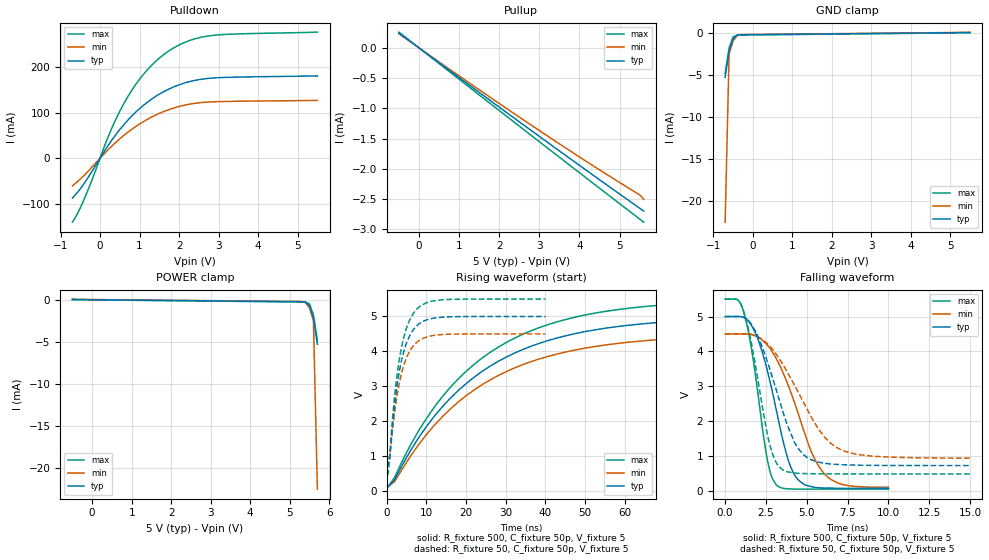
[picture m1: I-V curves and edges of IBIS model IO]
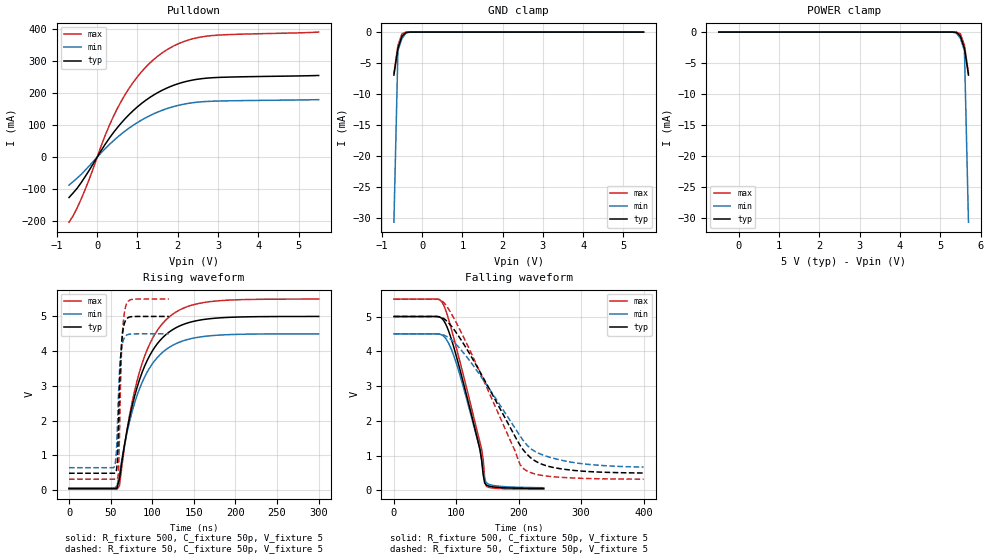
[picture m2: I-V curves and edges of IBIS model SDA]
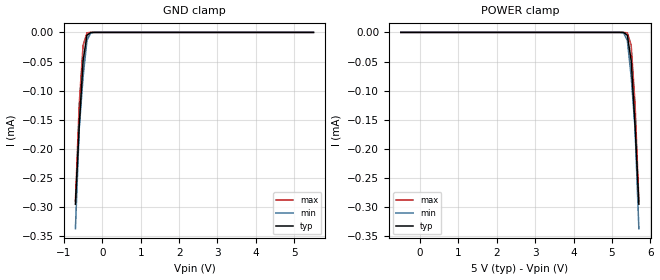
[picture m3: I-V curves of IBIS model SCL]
[IBIS Ver]   3.2
[Comment Char]   |_char
| VDD Nom: 5v, Min: 4.5v, Max: 5.5v
[File name]   pca9673_5v.ibs
[File Rev]   1
[Date]   08-25-2008
[Source]
[Notes]
[Disclaimer]
(C) Copyright 2007 NXP Semiconductors
All rights reserved
NXP Semiconductors (NXP) does not warrant that this model and any other
accompanying information (Model) accurately or fully represents the
operating characteristics and specifications of the semiconductor
products to which the Model relates.  Moreover, the Model is furnished
on an "as is" and with "all faults" basis, and without support or
warranty of any kind.  NXP disclaims all warranties, whether expressed
or implied or statutory, including without limitation all implied
warranties of non-infringement, merchantability and fitness for any
purpose, and those arising from a course of dealing or usage of trade.
NXP does not convey any license under its or any third party's patents,
copyrights or other intellectual property or proprietary rights.
You and your company assume any and all risks and liability arising out
of the application or use of the Model.
In no event shall NXP be liable for any direct, indirect, special,
consequential or incidental damages, however caused, whether in
warranty, contract or tort (including negligence), strict liability or
other legal theory, including, without limitation, for lost profits,
business interruption, or corruption or loss of data or information,
arising out of or in connection with the use of or the inability to use
the Model, even if NXP has been advised of the possibility of such
damages.
NXP provides the Model as a courtesy to our customers. You and your
company shall not distribute, convey, sell, or give the Model to anyone
else without receiving prior written permission from NXP.
NXP reserves the right to make changes without notice to the Model to
improve reliability, function, or design.
Please be aware that your receipt and subsequent use of the Model shall
serve as acceptance of these terms and conditions.  If you do not
accept these terms, return or destroy the Model immediately.
[Copyright]
2008
| SO24 package
[Component]   PCA9673D
Si_location Pin
Timing_location Pin
[Manufacturer]   NXP Semiconductors
[Package]
R_pkg   0.14   0.12   0.18
L_pkg   5.71n   3.95n   7.95n
C_pkg   1.01p   0.72p   1.49p
[Pin] signal_name   model_name   R_pin   L_pin   C_pin
1   INTb   INT   0.18   6.01n   0.97p
2   AD1   ADDR   0.14   7.94n   1.21p
3   RST   ADDR   0.16   7.06n   1.32p
4   P00   IO   0.18   6.01n   1.07p
5   P01   IO   0.14   4.98n   0.88p
6   P02   IO   0.13   4.30n   0.80p
7   P03   IO   0.12   3.95n   0.74p
8   P04   IO   0.12   3.95n   0.72p
9   P05   IO   0.13   4.30n   0.76p
10   P06   IO   0.14   4.98n   0.85p
11   P07   IO   0.18   6.01n   0.97p
12   VSS   GND   0.16   7.06n   1.20p
13   P10   IO   0.14   7.95n   1.45p
14   P11   IO   0.14   7.95n   1.49p
15   P12   IO   0.16   7.06n   1.32p
16   P13   IO   0.18   6.01n   1.07p
17   P14   IO   0.14   4.98n   0.88p
18   P15   IO   0.13   4.30n   0.80p
19   P16   IO   0.12   3.95n   0.74p
20   P17   IO   0.12   3.95n   0.72p
21   AD0   ADDR   0.13   4.30n   0.76p
22   SCL   SCL   0.14   4.98n   0.85p
23   SDA   SDA   0.18   6.01n   0.97p
24   VDD   POWER   0.16   7.06n   1.20p
| TSSOP24 package
[Component]   PCA9673PW
Si_location Pin
Timing_location Pin
[Manufacturer]   NXP Semiconductors
[Package]
R_pkg   52.70m   31.50m   67.00m
L_pkg   2.19n   1.32n   3.39n
C_pkg   0.48p   0.35p   0.93p
[Pin] signal_name   model_name   R_pin   L_pin   C_pin
1   INTb   INT   66.40m   2.36n   0.47p
2   AD1   ADDR   66.10m   3.39n   0.57p
3   RST   ADDR   67.00m   2.94n   0.59p
4   P00   IO   66.40m   2.36n   0.47p
5   P01   IO   47.10m   1.67n   0.40p
6   P02   IO   38.00m   1.44n   0.37p
7   P03   IO   31.50m   1.32n   0.35p
8   P04   IO   31.50m   1.32n   0.35p
9   P05   IO   38.00m   1.44n   0.37p
10   P06   IO   47.10m   1.67n   0.40p
11   P07   IO   66.40m   2.36n   0.47p
12   VSS   GND   67.00m   2.94n   0.59p
13   P10   IO   66.10m   3.39n   0.61p
14   P11   IO   66.20m   3.39n   0.61p
15   P12   IO   67.00m   2.94n   0.59p
16   P13   IO   66.50m   2.36n   0.47p
17   P14   IO   47.10m   1.67n   0.40p
18   P15   IO   38.00m   1.45n   0.37p
19   P16   IO   31.50m   1.32n   0.35p
20   P17   IO   31.50m   1.32n   0.35p
21   AD0   ADDR   38.00m   1.45n   0.37p
22   SCL   SCL   47.10m   1.67n   0.40p
23   SDA   SDA   66.50m   2.36n   0.47p
24   VDD   POWER   67.00m   2.94n   0.59p
| SSOP24
[Component]   PCA9673DB
Si_location Pin
Timing_location Pin
[Manufacturer]   NXP Semiconductors
[Package]
R_pkg   54.20m   39.70m   64.80m
L_pkg   2.55n   1.89n   3.58n
C_pkg   0.636p   0.52p   1.05p
[Pin] signal_name   model_name   R_pin   L_pin   C_pin
1   INTb   INT   63.00m   2.53n   0.58p
2   AD1   ADDR   61.20m   3.56n   0.70p
3   RST   ADDR   64.80m   3.10n   0.76p
4   P00   IO   63.00m   2.53n   0.60p
5   P01   IO   52.60m   2.17n   0.57p
6   P02   IO   43.90m   2.03n   0.56p
7   P03   IO   39.70m   1.89n   0.54p
8   P04   IO   39.70m   1.89n   0.52p
9   P05   IO   43.90m   2.03n   0.55p
10   P06   IO   52.60m   2.17n   0.56p
11   P07   IO   63.00m   2.53n   0.58p
12   VSS   GND   64.80m   3.10n   0.71p
13   P10   IO   61.20m   3.56n   1.01p
14   P11   IO   61.20m   3.56n   1.05p
15   P12   IO   64.80m   3.10n   0.80p
16   P13   IO   63.00m   2.53n   0.65p
17   P14   IO   52.60m   2.17n   0.59p
18   P15   IO   43.90m   2.03n   0.56p
19   P16   IO   39.70m   1.89n   0.54p
20   P17   IO   39.70m   1.89n   0.53p
21   AD0   ADDR   43.90m   2.03n   0.56p
22   SCL   SCL   52.60m   2.17n   0.57p
23   SDA   SDA   63.00m   2.53n   0.60p
24   VDD   POWER   64.80m   3.10n   0.76p
[Define Package Model]  HVQFN24
[Manufacturer]  ST-NXP Wireless
|[Simulated] Chris Hunat
|[Approved] Wayne Nunn, Roger Real
[OEM]  Unknown
[Description]  Full package model
[Number Of Pins]  23
[Pin Numbers]
pin1   | pin1 = lead1
pin2   | pin2 = lead2
pin3   | pin3 = lead3
pin4   | pin4 = lead4
pin5   | pin5 = lead5
pin6   | pin6 = lead6
pin7   | pin7 = lead7
pin8   | pin8 = lead8
pin9   | pin9 = lead9
pin10   | pin10 = lead10
pin11   | pin11 = lead11
pin12   | pin12 = lead12
pin13   | pin13 = lead13
pin14   | pin14 = lead14
pin15   | pin15 = lead15
pin17   | pin17 = lead17
pin18   | pin18 = lead18
pin19   | pin19 = lead19
pin20   | pin20 = lead20
pin21   | pin21 = lead21
pin22   | pin22 = lead22
pin23   | pin23 = lead23
pin24   | pin24 = lead24
[Model Data]
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[End Model Data]
[End Package Model]
[Define Package Model]  DHVQFN24
[Manufacturer]  ST-NXP Wireless
|[Simulated] Chris Hunat
|[Approved] Wayne Nunn, Roger Real
[OEM]  Unknown
[Description]  Full package model
[Number Of Pins]  24
[Pin Numbers]
|Pin Num   Terminal Name
1   | lead1:pin1
2   | lead2:pin2
3   | lead3:pin3
4   | lead4:pin4
5   | lead5:pin5
6   | lead6:pin6
7   | lead7:pin7
8   | lead8:pin8
9   | lead9:pin9
10   | lead10:pin10
11   | lead11:pin11
12   | lead12:pin12
13   | lead13:pin13
14   | lead14:pin14
15   | lead15:pin15
16   | lead16:pin16
17   | lead17:pin17
18   | lead18:pin18
19   | lead19:pin19
20   | lead20:pin20
21   | lead21:pin21
22   | lead22:pin22
23   | lead23:pin23
24   | lead24:pin24
[Model Data]
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[End Model Data]
[End Package Model]
| Models and submodels in the file (5): IO (I/O), SDA (I/O_open_drain), SCL (Input), ADDR (Input), INT (Open_drain)
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[Model]   IO
Model_type I/O
Vinh=3.5
Vinl=1.5
Vref=5
Vmeas=2.5
Rref=500
Cref=50p
C_comp   7p   6.8p   7.2p
[Model Spec]
Vinh   1.494   1.195   1.893
Vinl   1.023   0.854   1.563
[Temperature Range] 27   85   -40
[Voltage Range]   5   4.5   5.5
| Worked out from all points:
|   slope of the pulldown table from 0 to 0.75 V, typ, clamps not added: 8.52 ohm
|   slope of the pullup table from 0 to 0.75 V, typ, clamps not added: 2.03 kohm
|   GND clamp passes 1 mA (typ) near -0.52 V on its own axis
|   falling waveform, R_fixture 500, C_fixture 50p, V_fixture 5: 20-80 % time 1.51ns typ, 2.09ns min, 1ns max; typ from 5 V to 0.069 V
|   falling waveform, R_fixture 50, C_fixture 50p, V_fixture 5: 20-80 % time 1.82ns typ, 2.59ns min, 1.16ns max; typ from 5 V to 0.722 V
|   rising waveform, R_fixture 500, C_fixture 50p, V_fixture 5: 20-80 % time 28ns typ, 28.4ns min, 27.6ns max; typ from 0.069 V to 5 V
|   rising waveform, R_fixture 50, C_fixture 50p, V_fixture 5: 20-80 % time 3.48ns typ, 3.5ns min, 3.46ns max; typ from 0.722 V to 5 V
[Pullup]
-500mV    245.4uA    231.5uA    258.8uA
2.5V      -1.222mA   -1.144mA   -1.293mA
4.1V      -1.99mA    -1.846mA   -2.115mA
5.5V      -2.649mA   -2.43mA    -2.829mA
5.6V      -2.696mA   -2.5mA     -2.88mA
[Pulldown]
-700mV    -87.8mA    -60.93mA   -140.7mA
-600mV    -77.8mA    -53.55mA   -126.6mA
-400mV    -54.98mA   -37.53mA   -89.57mA
200mV     27.79mA    18.55mA    46.38mA
400mV     52.28mA    35.22mA    86.09mA
600mV     73.88mA    50.22mA    120.1mA
800mV     92.82mA    63.63mA    149.3mA
1.1V      116.7mA    80.88mA    185mA
1.6V      146.2mA    102.6mA    227.5mA
2.1V      164.7mA    116.2mA    253.5mA
2.7V      175.5mA    123.6mA    268.8mA
5.5V      181.5mA    127.5mA    277.8mA
[GND Clamp]
-700mV    -5.295mA   -22.53mA   -4.852mA
-600mV    -2.115mA   -2.495mA   -1.798mA
-500mV    -736.9uA   -981.7uA   -491.4uA
-400mV    -294uA     -348uA     -283.8uA
-200mV    -239.8uA   -212.7uA   -267.2uA
5.5V      23.22uA    77.99uA    169.3pA
[POWER Clamp]
-500mV    23.22uA    77.99uA    169.3pA
5.2V      -239.8uA   -212.7uA   -267.2uA
5.4V      -294uA     -348uA     -283.8uA
5.5V      -736.9uA   -981.7uA   -491.4uA
5.6V      -2.115mA   -2.495mA   -1.798mA
5.7V      -5.295mA   -22.53mA   -4.852mA
[Falling Waveform]
R_fixture=500
C_fixture=50p
V_fixture=5
V_fixture_min=4.5
V_fixture_max=5.5
0s        5V         4.5V       5.5V
1.111ns   4.983V     4.502V     5.168V
1.616ns   4.743V     4.484V     4.066V
2.626ns   3.367V     4.158V     790.5mV
3.131ns   2.318V     3.793V     169.1mV
3.737ns   1.08V      3.171V     57.77mV
4.242ns   460.2mV    2.53V      47.51mV
5.253ns   120.9mV    1.15V      45.47mV
6.061ns   77.51mV    494.8mV    45.06mV
10ns      69.28mV    98.13mV    44.81mV
[Falling Waveform]
R_fixture=50
C_fixture=50p
V_fixture=5
V_fixture_min=4.5
V_fixture_max=5.5
0s        5V         4.5V       5.5V
1.061ns   4.989V     4.502V     5.254V
1.818ns   4.606V     4.453V     3.701V
2.727ns   3.501V     4.156V     1.328V
3.485ns   2.343V     3.662V     611.1mV
4.242ns   1.394V     3.033V     507.3mV
4.848ns   1.014V     2.492V     493.1mV
6.061ns   792.3mV    1.553V     484.1mV
6.97ns    750.8mV    1.205V     482.4mV
15ns      722.3mV    933.8mV    481.5mV
[Rising Waveform]
R_fixture=500
C_fixture=50p
V_fixture=5
V_fixture_min=4.5
V_fixture_max=5.5
0s        69.03mV    93.83mV    44.8mV
2.02ns    311.4mV    260.4mV    380.9mV
6.061ns   1.155V     994.8mV    1.317V
10.1ns    1.85V      1.62V      2.083V
20.2ns    3.09V      2.74V      3.443V
32.32ns   3.954V     3.528V     4.383V
46.46ns   4.482V     4.014V     4.952V
62.63ns   4.768V     4.28V      5.258V
86.87ns   4.931V     4.433V     5.429V
200ns     5V         4.5V       5.5V
[Rising Waveform]
R_fixture=50
C_fixture=50p
V_fixture=5
V_fixture_min=4.5
V_fixture_max=5.5
0s        722.2mV    930.6mV    481.5mV
404ps     722.2mV    930.6mV    481.8mV
808.1ps   917.4mV    980.2mV    958.8mV
2.02ns    2.46V      2.237V     2.7V
2.828ns   3.158V     2.852V     3.473V
3.636ns   3.663V     3.306V     4.036V
5.253ns   4.304V     3.874V     4.738V
7.677ns   4.738V     4.264V     5.215V
14.14ns   4.981V     4.483V     5.479V
40ns      5V         4.5V       5.5V
[Ramp]
R_load=500
dV/dt_r   6.301E-1/1.024E-9   5.382E-1/1.436E-9   7.243E-1/7.748E-10
dV/dt_f   2.959E+0/3.658E-10   2.644E+0/6.004E-10   3.273E+0/2.083E-10
|[End   IO
| [End   SDA
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[Model]   SDA
Model_type I/O_open_drain
Vinh=3.5
Vinl=1.5
Vref=5
Vmeas=2.5
Rref=1k
Cref=50p
C_comp   6p   5.8p   6.2p
[Model Spec]
[Temperature Range] 27   85   -40
[Voltage Range]   5   4.5   5.5
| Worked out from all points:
|   slope of the pulldown table from 0 to 0.75 V, typ, clamps not added: 5.88 ohm
|   GND clamp passes 1 mA (typ) near -0.52 V on its own axis
|   falling waveform, R_fixture 500, C_fixture 50p, V_fixture 5: 20-80 % time 41.4ns typ, 39.1ns min, 45.5ns max; typ from 5 V to 0.053 V
|   falling waveform, R_fixture 50, C_fixture 50p, V_fixture 5: 20-80 % time 83.3ns typ, 86.1ns min, 78.4ns max; typ from 5 V to 0.498 V
|   rising waveform, R_fixture 500, C_fixture 50p, V_fixture 5: 20-80 % time 35.3ns typ, 35.4ns min, 35.3ns max; typ from 0.047 V to 5 V
|   rising waveform, R_fixture 50, C_fixture 50p, V_fixture 5: 20-80 % time 3.87ns typ, 4.13ns min, 3.67ns max; typ from 0.488 V to 5 V
[Pulldown]
-700mV    -126.5mA   -87.42mA   -203.7mA
-600mV    -112.5mA   -77.06mA   -184.2mA
-400mV    -80.24mA   -54.43mA   -131.7mA
-200mV    -41.6mA    -27.72mA   -69.88mA
200mV     40.47mA    26.71mA    68.47mA
500mV     92.1mA     61.87mA    152mA
700mV     121.1mA    82.16mA    197.1mA
1V        157.3mA    108.2mA    251.7mA
1.5V      201.5mA    140.8mA    315.4mA
2V        229.2mA    161.5mA    353.8mA
2.6V      245.5mA    173.1mA    376.2mA
5.5V      255.4mA    179.8mA    391.2mA
[GND Clamp]
-700mV    -6.935mA   -30.66mA   -6.593mA
-600mV    -2.591mA   -2.99mA    -2.148mA
-500mV    -653.7uA   -1.019mA   -278.6uA
-400mV    -54.45uA   -160.3uA   -7.607uA
-200mV    -25.65nA   -197.3nA   -667.7pA
5.5V      311.2pA    571.6pA    286.3pA
[POWER Clamp]
-500mV    311.2pA    571.6pA    286.3pA
5.2V      -25.65nA   -197.3nA   -667.7pA
5.4V      -54.45uA   -160.3uA   -7.607uA
5.5V      -653.7uA   -1.019mA   -278.6uA
5.6V      -2.591mA   -2.99mA    -2.148mA
5.7V      -6.935mA   -30.66mA   -6.593mA
[Falling Waveform]
R_fixture=500
C_fixture=50p
V_fixture=5
V_fixture_min=4.5
V_fixture_max=5.5
0s        5V         4.5V       5.5V
70.3ns    4.998V     4.499V     5.498V
80ns      4.877V     4.428V     5.315V
101.8ns   3.74V      3.549V     3.978V
135.8ns   1.343V     1.314V     1.536V
140.6ns   855mV      873.4mV    1.176V
143ns     443.6mV    560.4mV    887.1mV
145.5ns   207.4mV    315.8mV    345.9mV
147.9ns   153.8mV    222.2mV    126mV
240ns     53.13mV    74.44mV    33.52mV
[Falling Waveform]
R_fixture=50
C_fixture=50p
V_fixture=5
V_fixture_min=4.5
V_fixture_max=5.5
0s        5V         4.5V       5.5V
68.69ns   4.999V     4.499V     5.5V
80.81ns   4.929V     4.46V      5.384V
96.97ns   4.609V     4.247V     4.921V
121.2ns   3.93V      3.732V     4.047V
202ns     1.3V       1.568V     742.3mV
210.1ns   1.1V       1.366V     590.8mV
230.3ns   805.4mV    1.08V      452.3mV
262.6ns   633.3mV    890.4mV    379.8mV
400ns     498.2mV    668.4mV    321.2mV
[Rising Waveform]
R_fixture=500
C_fixture=50p
V_fixture=5
V_fixture_min=4.5
V_fixture_max=5.5
0s        46.79mV    64.38mV    29.93mV
54.55ns   46.79mV    65.45mV    29.93mV
57.58ns   57.12mV    114mV      29.92mV
60.61ns   321.9mV    447.6mV    122.5mV
72.73ns   2.087V     1.974V     2.147V
84.85ns   3.189V     2.928V     3.418V
103ns     4.114V     3.729V     4.482V
124.2ns   4.615V     4.165V     5.059V
172.7ns   4.943V     4.45V      5.435V
300ns     5V         4.5V       5.5V
[Rising Waveform]
R_fixture=50
C_fixture=50p
V_fixture=5
V_fixture_min=4.5
V_fixture_max=5.5
0s        488mV      647.3mV    317.3mV
53.33ns   488mV      647.7mV    317.3mV
55.76ns   490.7mV    799.3mV    317.3mV
58.18ns   820.9mV    1.85V      324.3mV
59.39ns   1.777V     2.723V     469.6mV
60.61ns   2.939V     3.383V     1.502V
61.82ns   3.71V      3.803V     2.994V
64.24ns   4.503V     4.231V     4.534V
67.88ns   4.882V     4.436V     5.27V
120ns     5V         4.5V       5.5V
[Ramp]
R_load=500
dV/dt_r   2.972E+0/1.196E-9   2.957E+0/1.676E-9   2.984E+0/8.187E-10
dV/dt_f   2.948E+0/4.154E-8   2.907E+0/4.355E-8   2.973E+0/4.126E-8
|[End   SDA
| [End   SCL
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[Model]   SCL
Model_type Input
Vinh=3.5
Vinl=1.5
C_comp   5p   4.8p   5.2p
[Model Spec]
Vinh   2.31   1.61   3.85
Vinl   0.99   0.69   1.65
[Temperature Range] 27   85   -40
[Voltage Range]   5   4.5   5.5
[GND Clamp]
-700mV    -295uA     -337uA     -289.5uA
-600mV    -158.8uA   -164.3uA   -122uA
-500mV    -48.62uA   -75.94uA   -22.35uA
-400mV    -4.926uA   -13.83uA   -710.6nA
-300mV    -138.4nA   -722.3nA   -7.551nA
5.5V      13.38pA    37.84pA    11.03pA
[POWER Clamp]
-500mV    13.38pA    37.84pA    11.03pA
5.3V      -138.4nA   -722.3nA   -7.551nA
5.4V      -4.926uA   -13.83uA   -710.6nA
5.5V      -48.62uA   -75.94uA   -22.35uA
5.6V      -158.8uA   -164.3uA   -122uA
5.7V      -295uA     -337uA     -289.5uA
